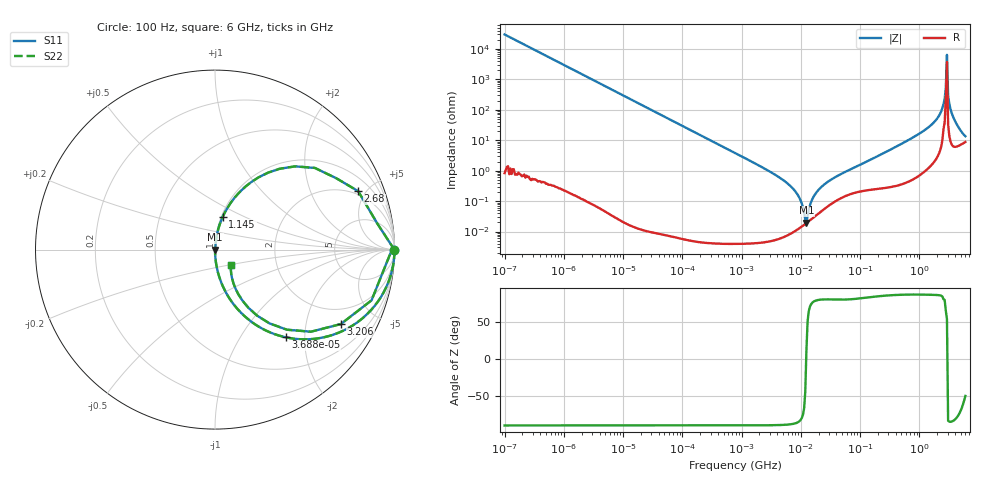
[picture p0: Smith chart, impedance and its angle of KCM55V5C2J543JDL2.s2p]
!Murata Part Number: KCM55V5C2J543JDL2
!These Parameters are Measured in Series Mode Connection
!Data Generated on Mar 13, 2026
!  o--ll--o
!Port1  Port2
!  o------o
!Operation Temp=25[degC], DC Bias Voltage=0[V]
!Freq. Start=100[Hz] Stop=6[GHz] 401[Steps]
# Hz S RI R 50
!Freq.(Hz) S11(Real) S11(Imag) S21(Real) S21(Imag) S12(Real) S12(Imag) S22(Real) S22(Imag)
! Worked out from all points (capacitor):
!   401 points, 100 Hz to 6 GHz, reference 50 ohm
!   read as one part in series: C = 53.5 nF near 109 Hz
!   lowest |Z| = 19.4 mohm at 12.44 MHz (marker M1)
!   series resonance near 12.34 MHz, so ESL is about 3.1 nH
!   S11 on the Smith chart (normalised r, x): 100 Hz: open; 36.88 kHz: 1.00, -1.61; 1.145 GHz: 1.02, +0.39; 2.68 GHz: 1.75, +4.43; 3.206 GHz: 1.29, -3.17; 6 GHz: 1.17, -0.21
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100  1 -0.00336  1.14e-05 0.00336  1.14e-05 0.00336  1 -0.00336
2008  0.9955 -0.0672  0.00454 0.0672  0.00454 0.0672  0.9955 -0.0672
11009  0.8795 -0.3255  0.1205 0.3255  0.1205 0.3255  0.8795 -0.3255
36880  0.3941 -0.4886  0.6059 0.4886  0.6059 0.4886  0.3941 -0.4886
40335  0.3523 -0.4776  0.6477 0.4776  0.6477 0.4776  0.3523 -0.4776
112960  0.0649 -0.2462  0.9351 0.2462  0.9351 0.2462  0.0649 -0.2462
774597  0.0015 -0.0382  0.9985 0.0382  0.9985 0.0382  0.0015 -0.0382
6353432  9.15e-05 -0.00343  0.9999 0.00343  0.9999 0.00343  9.15e-05 -0.00343
9090158  0.000124 -0.00148  0.9999 0.00148  0.9999 0.00148  0.000124 -0.00148
1.243624e7  0.00019 3.89e-05  0.9998 -3.89e-05  0.9998 -3.89e-05  0.00019 3.89e-05
1.555665e7  0.000269 0.0011  0.9997 -0.0011  0.9997 -0.0011  0.000269 0.0011
3.184506e7  0.000804 0.0049  0.9992 -0.0049  0.9992 -0.0049  0.000804 0.0049
3.124326e8  0.00502 0.0466  0.995 -0.0466  0.995 -0.0466  0.00502 0.0466
1.144649e9  0.0439 0.1844  0.9561 -0.1844  0.9561 -0.1844  0.0439 0.1844
2.240541e9  0.3603 0.4505  0.6397 -0.4505  0.6397 -0.4505  0.3603 0.4505
2.562649e9  0.676 0.3974  0.324 -0.3974  0.324 -0.3974  0.676 0.3974
2.679998e9  0.7976 0.3255  0.2024 -0.3255  0.2024 -0.3255  0.7976 0.3255
2.931063e9  0.9907 0.0125  0.00926 -0.0125  0.00926 -0.0125  0.9907 0.0125
3.205649e9  0.701 -0.415  0.299 0.415  0.299 0.415  0.701 -0.415
3.352442e9  0.5342 -0.4575  0.4658 0.4575  0.4658 0.4575  0.5342 -0.4575
3.666503e9  0.3029 -0.4108  0.6971 0.4108  0.6971 0.4108  0.3029 -0.4108
6e9  0.0886 -0.0869  0.9114 0.0869  0.9114 0.0869  0.0886 -0.0869
